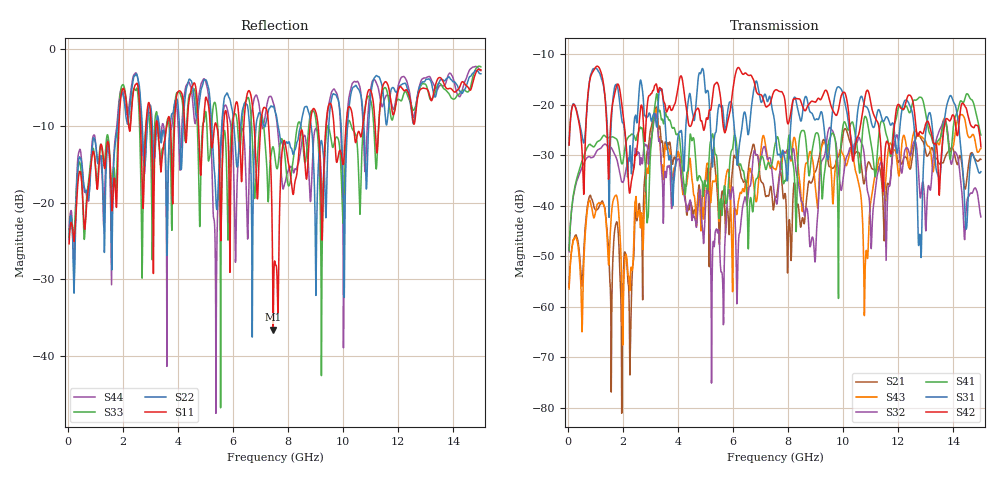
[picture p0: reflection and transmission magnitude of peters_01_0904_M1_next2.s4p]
# MHZ S RI R 50.00
! FREQ  S11  S12  S13  S14
!  S21  S22  S23  S24
!  S31  S32  S33  S34
!  S41  S42  S43  S44
!  REAL  IMAG  REAL  IMAG  REAL  IMAG  REAL  IMAG
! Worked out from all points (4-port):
!   1496 points, 50 MHz to 15 GHz, reference 50 ohm
!   strongest paths, dB at 50 MHz, 3.79 GHz, 7.53 GHz, 11.27 GHz, 15 GHz:
!     S42: -28.0, -21.1, -17.2, -23.7, -28.4
!     S31: -27.9, -37.4, -24.5, -21.1, -33.3
!     S41: -48.9, -24.6, -27.8, -27.6, -26.0
!     S32: -49.1, -39.3, -38.4, -33.3, -42.2
!     S43: -56.5, -34.7, -32.8, -31.5, -28.7
!     S21: -56.1, -31.6, -38.3, -32.5, -30.9
!   lowest |S11| = -36.5 dB at 7.46 GHz (marker M1), VSWR 1.03, Z = 49.6 + j1.42 ohm
!   |S11| at or under -10 dB: start of sweep to 1.858 GHz; 7.293 GHz to 8.799 GHz (1.507 GHz wide, 18.7 % of centre); 9.666 GHz to 10.1 GHz (437.3 MHz wide, 4.42 % of centre)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
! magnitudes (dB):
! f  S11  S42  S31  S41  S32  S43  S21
! 50 MHz  -25.3  -28.0  -27.9  -48.9  -49.1  -56.5  -56.1
! 2.26 GHz  -10.7  -37.3  -28.2  -26.2  -31.1  -56.6  -73.5
! 3.18 GHz  -11.0  -16.1  -22.7  -19.5  -21.9  -21.5  -21.0
! 5.61 GHz  -15.1  -22.4  -20.3  -41.5  -53.7  -40.6  -37.1
! 7.46 GHz  -36.5  -17.7  -21.8  -30.2  -35.8  -32.6  -40.8
! 10.82 GHz  -7.0  -17.8  -20.4  -22.4  -33.5  -49.7  -33.8
! 15 GHz  -2.7  -28.4  -33.3  -26.0  -42.2  -28.7  -30.9
